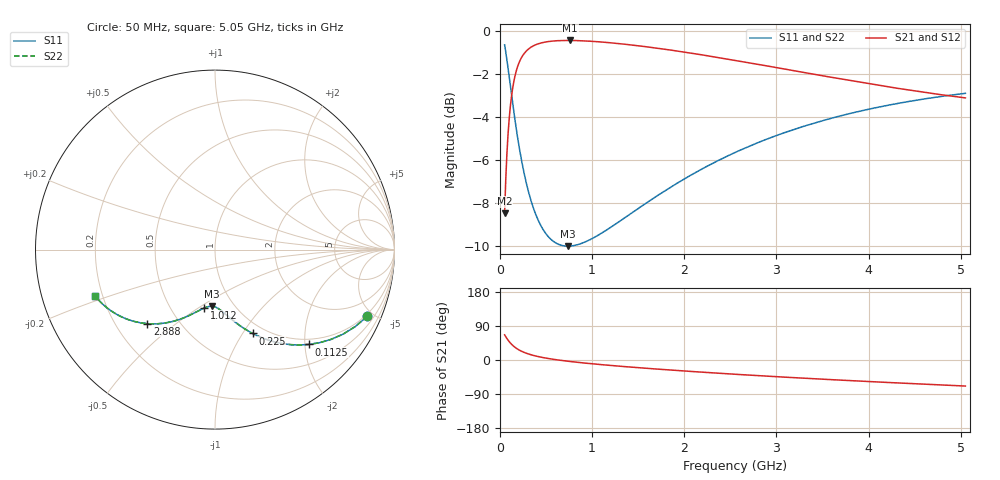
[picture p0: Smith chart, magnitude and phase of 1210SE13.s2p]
! AVX Thin Film Operation		Date: August 2001
! Description: Accu-P® Series, Thin Film, SMD, RF Capacitor
! Part Number: 12101J130FBT
! 50 MHz  -  5.05 GHz
! Serial Measurements
# mhz S db R 50
!	S11		S21		S12		S22
!	dB	Phase	dB	Phase	dB	Phase	dB	Phase
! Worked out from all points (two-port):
!   401 points, 50 MHz to 5.05 GHz, reference 50 ohm
!   highest |S21| = -0.46 dB at 762.5 MHz (marker M1); lowest = -8.5 dB at 50 MHz (marker M2)
!   |S21| within 3 dB of the highest: 113.9 MHz to end of sweep
!   lowest |S11| = -10.0 dB at 737.5 MHz (marker M3), VSWR 1.92, Z = 39.6 - j27.8 ohm
!   |S11| at or under -10 dB: 707.1 MHz to 768.8 MHz (61.61 MHz wide, 8.35 % of centre)
!   |S22| runs from -10.0 to -0.7 dB; largest |S21 - S12| = 0
!   S11 on the Smith chart (normalised r, x): 50 MHz: 0.88, -4.63; 112.5 MHz: 0.88, -2.09; 225 MHz: 0.88, -1.11; 1.012 GHz: 0.73, -0.53; 2.888 GHz: 0.33, -0.40; 5.05 GHz: 0.17, -0.18
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50  -0.66 -23.6  -8.49 66.4  -8.49 66.4  -0.66 -23.6
75  -1.36 -33.4  -5.71 56.6  -5.71 56.6  -1.36 -33.4
87.5  -1.75 -37.7  -4.80 52.3  -4.80 52.3  -1.75 -37.7
112.5  -2.56 -45.2  -3.51 44.8  -3.51 44.8  -2.56 -45.2
137.5  -3.38 -51.4  -2.67 38.6  -2.67 38.6  -3.38 -51.4
162.5  -4.15 -56.5  -2.11 33.5  -2.11 33.5  -4.15 -56.5
225  -5.82 -65.9  -1.32 24.1  -1.32 24.1  -5.82 -65.9
300  -7.33 -73.4  -0.89 16.6  -0.89 16.6  -7.33 -73.4
400  -8.66 -80.2  -0.64 9.8  -0.64 9.8  -8.66 -80.2
550  -9.68 -87.0  -0.50 2.9  -0.50 2.9  -9.68 -87.0
737.5  -10.01 -93.2  -0.46 -3.3  -0.46 -3.3  -10.01 -93.2
762.5  -10.00 -93.9  -0.46 -4.0  -0.46 -4.0  -10.00 -93.9
887.5  -9.87 -97.3  -0.47 -7.3  -0.47 -7.3  -9.87 -97.3
1012.5  -9.63 -100.2  -0.50 -10.3  -0.50 -10.3  -9.63 -100.2
1350  -8.70 -107.4  -0.63 -17.4  -0.63 -17.4  -8.70 -107.4
1725  -7.62 -114.3  -0.83 -24.3  -0.83 -24.3  -7.62 -114.3
2125  -6.58 -121.0  -1.08 -31.0  -1.08 -31.0  -6.58 -121.0
2550  -5.66 -127.6  -1.38 -37.6  -1.38 -37.6  -5.66 -127.6
2887.5  -5.05 -132.4  -1.63 -42.5  -1.63 -42.5  -5.05 -132.5
3387.5  -4.32 -139.2  -2.01 -49.2  -2.01 -49.2  -4.32 -139.2
4225  -3.45 -149.4  -2.62 -59.5  -2.62 -59.5  -3.45 -149.4
5050  -2.91 -158.7  -3.12 -68.7  -3.12 -68.7  -2.91 -158.7
